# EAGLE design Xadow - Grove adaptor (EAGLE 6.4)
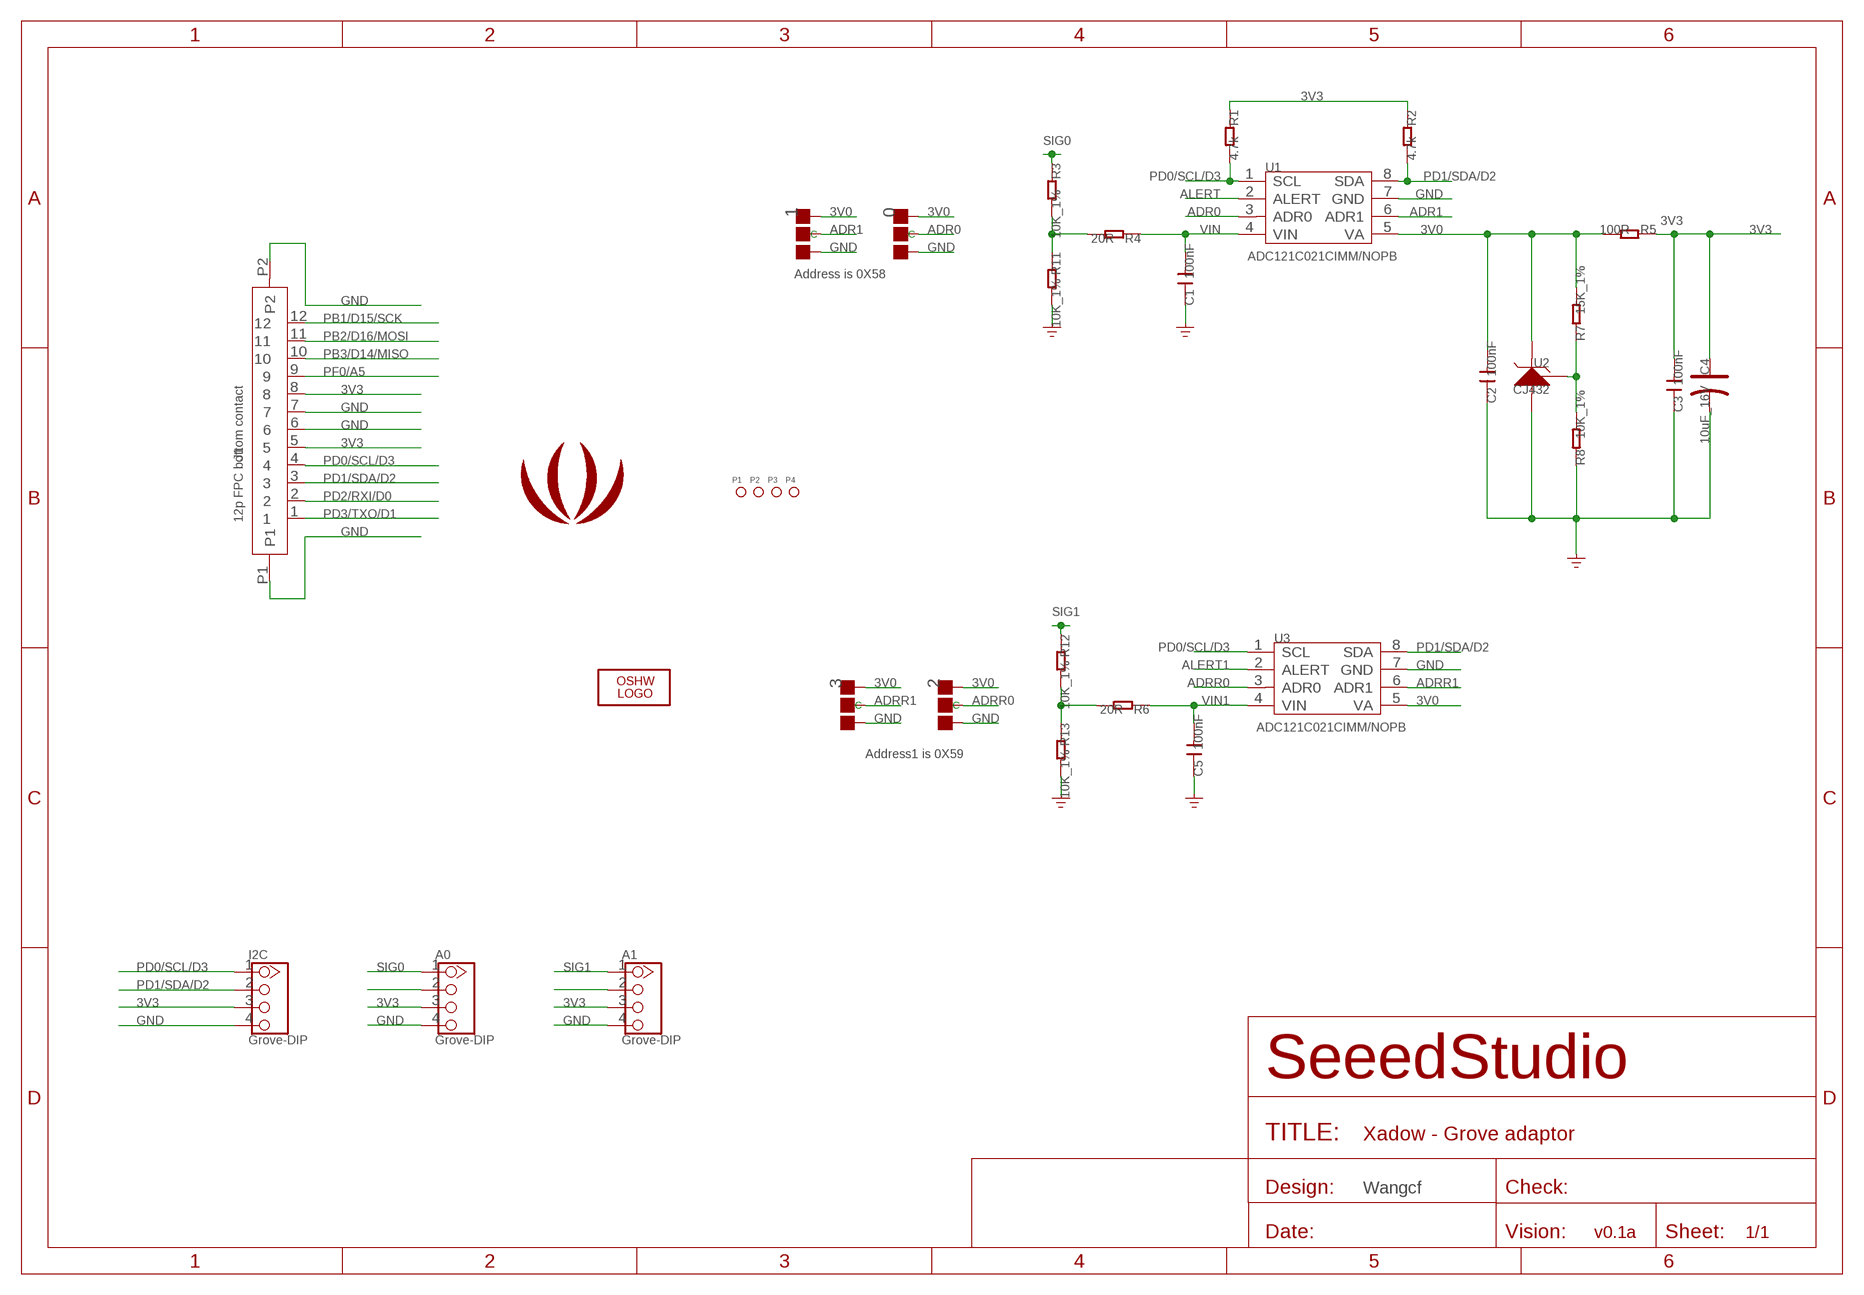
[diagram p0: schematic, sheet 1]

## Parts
0  DNP  PAD-JUMPER-3P-40*40  [3P-SMD-4.1X1.5]
1  DNP  PAD-JUMPER-3P-40*40  [3P-SMD-4.1X1.5]
2  DNP  PAD-JUMPER-3P-40*40  [3P-SMD-4.1X1.5]
3  DNP  PAD-JUMPER-3P-40*40  [3P-SMD-4.1X1.5]
A0  Grove-DIP  TWIG-2.0-LEADED  [4P-LEADED-2.0]
A1  Grove-DIP  TWIG-2.0-LEADED  [4P-LEADED-2.0]
C1  100nF  C-0603  [C0603]
C2  100nF  C-0603  [C0603]
C3  100nF  C-0603  [C0603]
C4  10uF_16V  CAP-AVX-A  [AVX-A]
C5  100nF  C-0603  [C0603]
I2C  Grove-DIP  TWIG-2.0-LEADED  [4P-LEADED-2.0]
J1  12p FPC bottom contact  FPC052002-12LT  [12P-0.5]
LOGO2  LOGO-OSHW-FILLX0100-NT  [OSHW_FILLX100_NOTEXT]
P1  PAD-MARK  [ROUND-MARK-1.0]
P2  PAD-MARK  [ROUND-MARK-1.0]
P3  PAD-MARK  [ROUND-MARK-1.0]
P4  PAD-MARK  [ROUND-MARK-1.0]
R1  4.7k  R-0603  [R0603]
R2  4.7k  R-0603  [R0603]
R3  10K_1%  R-0603  [R0603]
R4  20R  R-0603  [R0603]
R5  100R  R-0603  [R0603]
R6  20R  R-0603  [R0603]
R7  15K_1%  R-0603  [R0603]
R8  10K_1%  R-0603  [R0603]
R11  10K_1%  R-0603  [R0603]
R12  10K_1%  R-0603  [R0603]
R13  10K_1%  R-0603  [R0603]
U1  ADC121C021CIMM/NOPB  ADC121C021'CIMM/NP8'  [MSOP8]
U2  CJ432  REFERENCE-SOURCE  [SOT23]
U3  ADC121C021CIMM/NOPB  ADC121C021'CIMM/NP8'  [MSOP8]
U$7  LOGO-SEEEDSTUDIO-SMALL-SILK  [SMALL_SEEED_LOGO]

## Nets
3V0: 0.11(R) 1.11(R) 2.11(R) 3.11(R) C2.2 R5.2 R7.2 U1.5(VA) U2.2(K) U3.5(VA)
3V3: A0.3 A1.3 C3.2 C4.+ I2C.3 J1.5 J1.8 R1.1 R2.1 R5.1
ADR0: 0.MM(C) U1.3(ADR0)
ADR1: 1.MM(C) U1.6(ADR1)
ADRR0: 2.MM(C) U3.3(ADR0)
ADRR1: 3.MM(C) U3.6(ADR1)
ALERT: U1.2(ALERT)
ALERT1: U3.2(ALERT)
GND: 0.00(L) 1.00(L) 2.00(L) 3.00(L) A0.4 A1.4 C1.1 C2.1 C3.1 C4.- C5.1 I2C.4 J1.6 J1.7 J1.P1 J1.P2 R8.1 R11.2 R13.2 U1.7(GND) U2.3(A) U3.7(GND)
N$1: R7.1 R8.2 U2.1(R)
N$2: R3.2 R4.2 R11.1
N$3: R6.2 R12.2 R13.1
N$4: A0.2
N$5: A1.2
PB1/D15/SCK: J1.12
PB2/D16/MOSI: J1.11
PB3/D14/MISO: J1.10
PD0/SCL/D3: I2C.1 J1.4 R1.2 U1.1(SCL) U3.1(SCL)
PD1/SDA/D2: I2C.2 J1.3 R2.2 U1.8(SDA) U3.8(SDA)
PD2/RXI/D0: J1.2
PD3/TXO/D1: J1.1
PF0/A5: J1.9
SIG0: A0.1 R3.1
SIG1: A1.1 R12.1
VIN: C1.2 R4.1 U1.4(VIN)
VIN1: C5.2 R6.1 U3.4(VIN)

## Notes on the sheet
- 3V3
- Address is 0X58
- Address1 is 0X59
- Wangcf
- v0.1a

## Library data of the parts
0 1-3 = Discrete:PAD-JUMPER-3P; PARTNO: DNP
A0 A1 I2C = Connector:TWIG-2.0-LEADED
C1-C3 C5 = Discrete:C*: Ceramic Capacitors
C4 = Discrete1:CAP*: Electrolytic Capacitors,Tantalum Capacitors and Super Capacitors
J1 = template:FPC052002-12LT
LOGO2 = Logo:LOGO-OSHW-FILL; PARTNO: DNP
P1-P4 = Discrete:PAD-MARK; PARTNO: DNP
R1-R8 R11-R13 = Discrete:R*
U1 U3 = IC:ADC121C021: ADC121C021/ADC121C021Q/ADC121C027 I2C-Compatible, 12-Bit Analog-to-Digital Converter with Alert Function
U2 = For_Test_Albert_v6:REFERENCE-SOURCE: CJ432,AZ432 or other Adjustable Reference Source
U$7 = Logo:LOGO-SEEEDSTUDIO; PARTNO: DNP

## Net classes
0 default: width 0.152 mm, drill 0.305 mm, clearance 0.152 mm
1 GND: width 0.152 mm, drill 0.305 mm, clearance 0.152 mm to class 0, clearance 0.152 mm
3 usbvcc: width 0.203 mm, drill 0.305 mm, clearance 0.203 mm

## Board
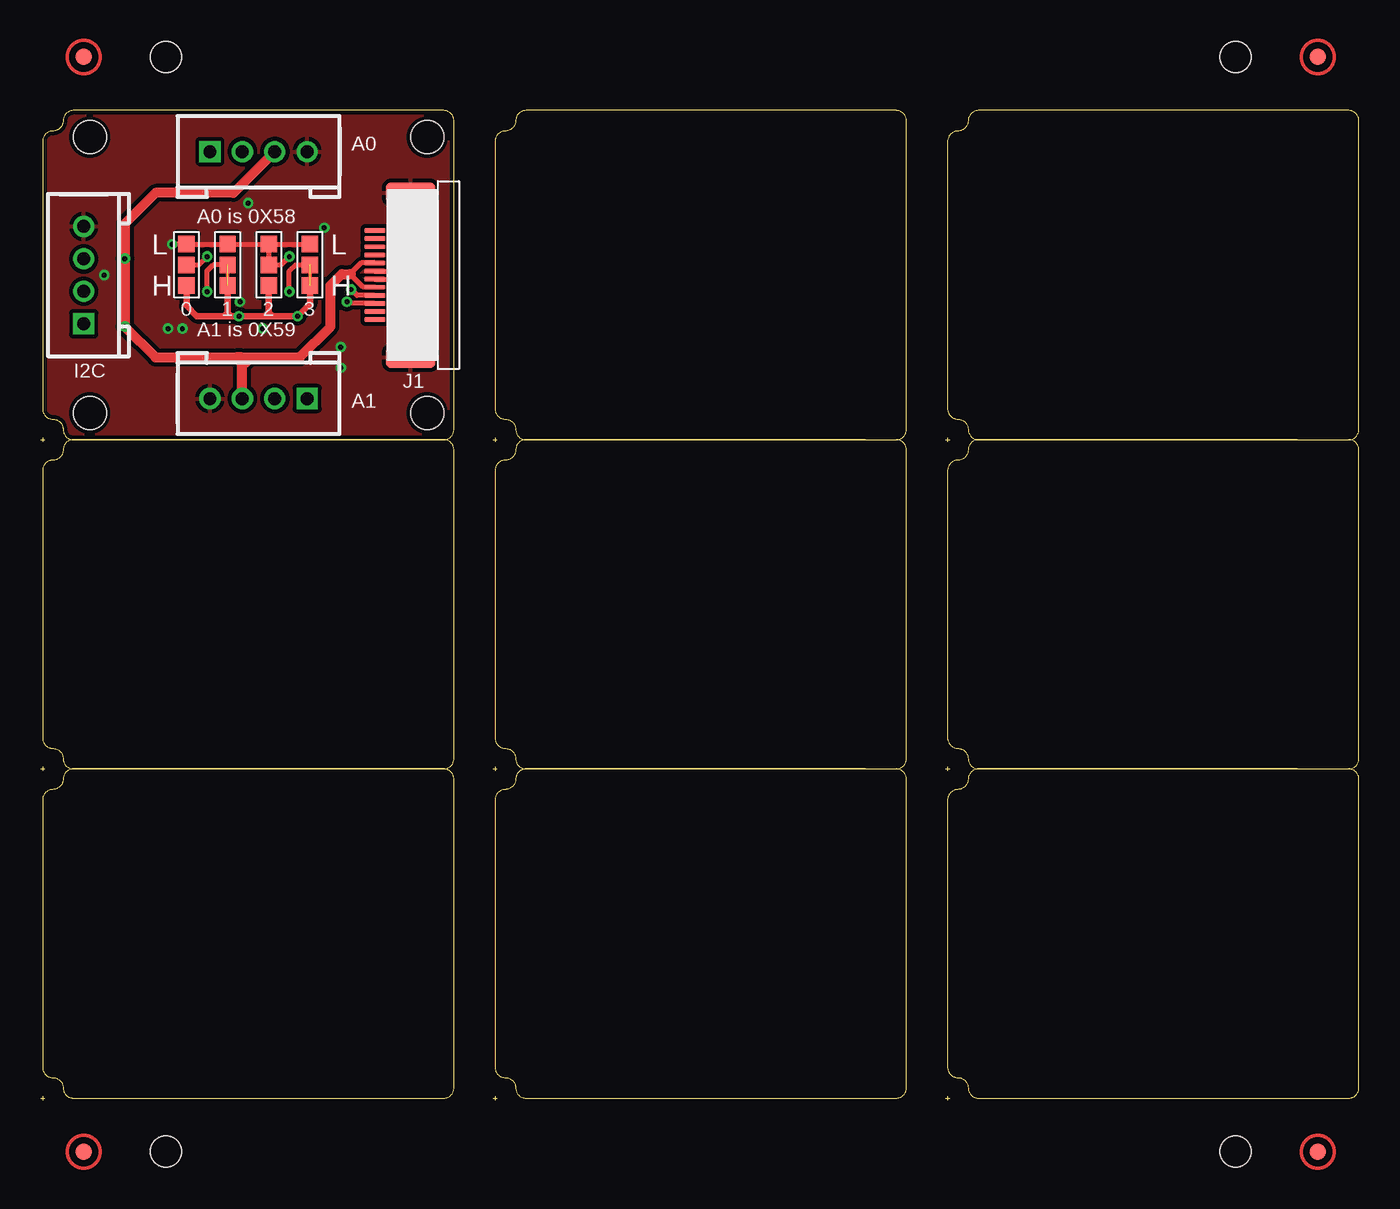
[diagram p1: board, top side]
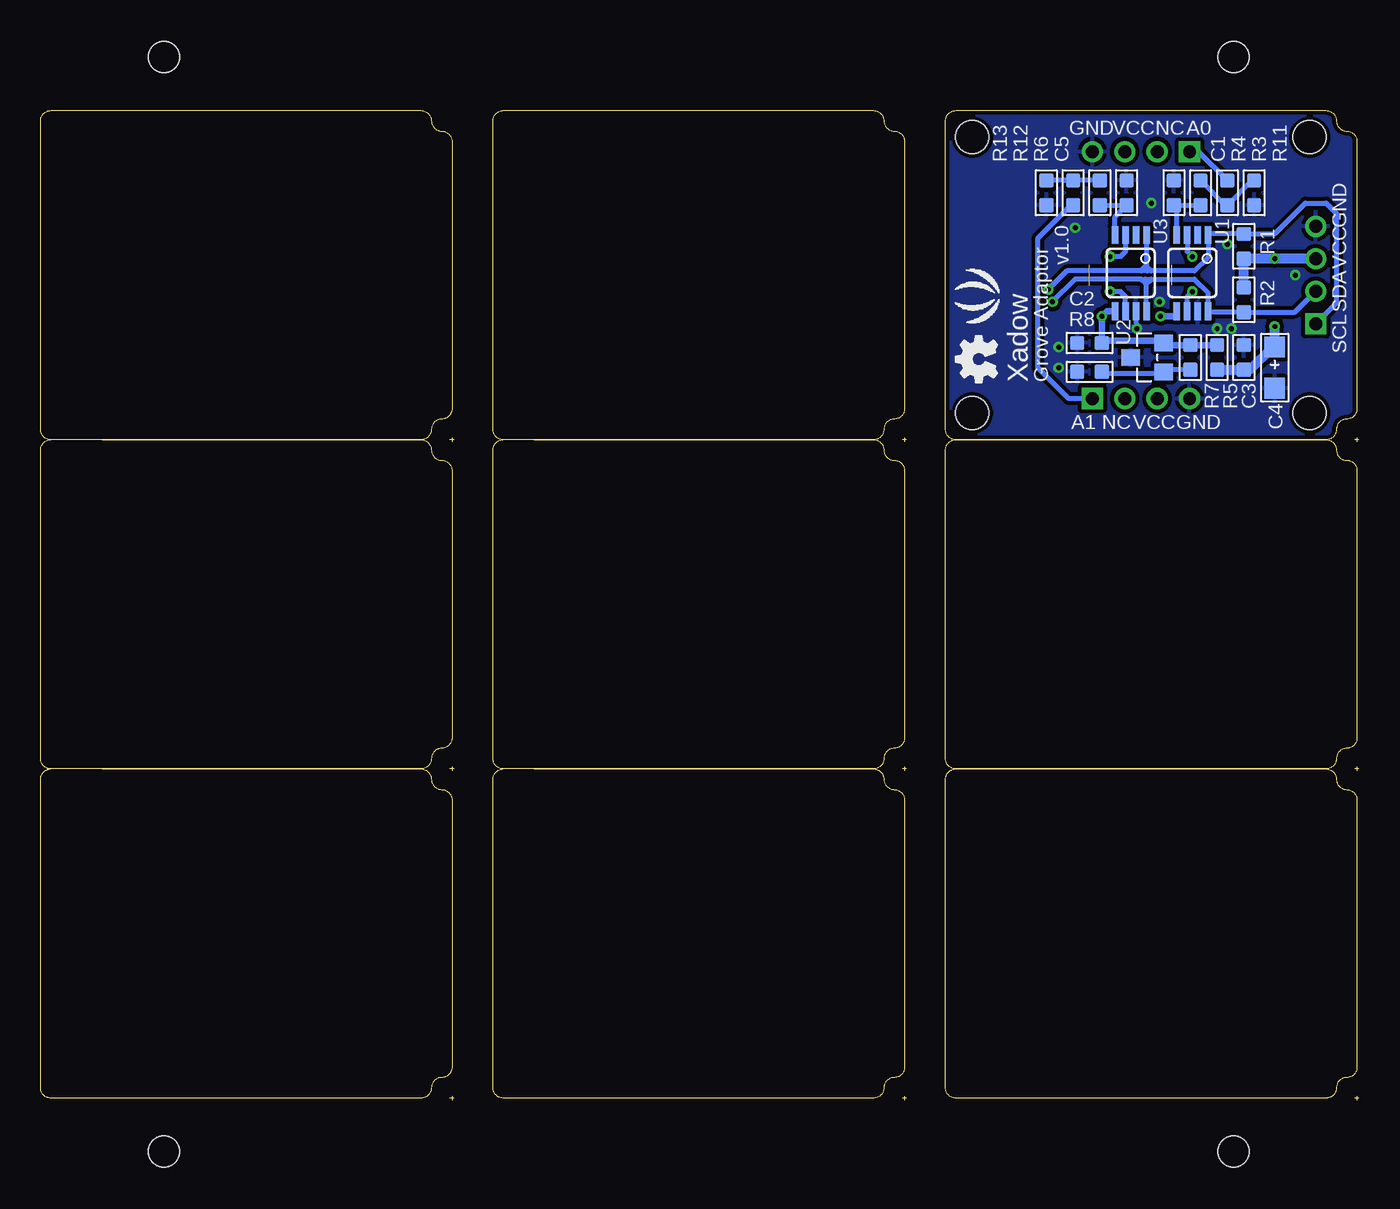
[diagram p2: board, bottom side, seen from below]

Size 81.41 x 61.09 mm. Coordinates in mm from the lower left corner, seen from the top.
Outline: 181 segments
Copper layers (1*16): Top 0.035mm / dielectric 1.5mm / Bottom 0.035mm
Design rules "SeeedStudio_rule_no_angle_090911 *": minimum track width 6mil, minimum drill 12mil, track to track 6mil, track to pad 6mil, pad to pad 6mil, via to via 6mil, smd to smd 0mil, copper to edge 10mil, drill to drill 10mil, minimum pad ring 10mil, minimum via ring 6mil, stop-mask expansion 2mil, vias tented up to drill 25mil, thermal gap 10mil
Holes 2.03 mm at 3.05,42.42 3.05,59.44 23.88,59.44 23.88,42.42
Holes 1.91 mm at 73.79,64.39 7.75,64.39 7.75,-3.17 73.79,-3.17
tRestrict: area 20.3,50.9 to 21,51

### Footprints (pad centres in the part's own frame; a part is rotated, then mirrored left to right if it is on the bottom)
3P-SMD-4.1X1.5 = smd 1.016 x 1.016: 00 -1.27,0; 11 1.27,0; MM 0,0
4P-LEADED-2.0 = drill 0.8 pad 1.27 square: 1 -3,0 | drill 0.8 pad 1.27: 2 -1,0; 3 1,0; 4 3,0
C0603 = smd 0.889 x 0.889: 1 -0.762,0; 2 0.762,0
AVX-A = smd 1.27 x 1.27: + -1.27,0; - 1.27,0
12P-0.5 = smd 0.3 x 1.3: 1 -2.75,2.35; 2 -2.25,2.35; 3 -1.75,2.35; 4 -1.25,2.35; 5 -0.75,2.35; 6 -0.25,2.35; 7 0.25,2.35; 8 0.75,2.35; 9 1.25,2.35; 10 1.75,2.35; 11 2.25,2.35; 12 2.75,2.35 | smd 1.27 x 3.048: P1 -5.08,0.127; P2 5.08,0.127
ROUND-MARK-1.0 = smd 1.016 x 1.016: P$1 0,0
R0603 = smd 0.889 x 0.889: 1 -0.762,0; 2 0.762,0
MSOP8 = smd 1.1 x 0.4: 1 -2.477,0.975; 2 -2.477,0.325; 3 -2.477,-0.325; 4 -2.477,-0.975; 5 2.223,-0.975; 6 2.223,-0.325; 7 2.223,0.325; 8 2.223,0.975
SOT23 = smd 1.016 x 1.143: 1 -0.889,-1.016; 2 0.889,-1.016; 3 0,1.016

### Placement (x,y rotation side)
0  9.02,51.56 270 top
1  11.56,51.56 270 top
2  14.1,51.56 270 top
3  16.64,51.56 270 top
A0  13.46,58.55 0 top
A1  13.46,43.31 180 top
C1  11.43,56.01 270 bottom
C2  16.64,46.74 0 bottom
C3  7.11,45.85 270 bottom
C4  5.21,45.21 270 bottom
C5  14.35,56.01 270 bottom
I2C  2.67,50.93 90 top
J1  22.99,50.93 90 top
LOGO2  22.35,44.32 90 bottom
P1  not placed on the board
P2  not placed on the board
P3  not placed on the board
P4  not placed on the board
R1  7.11,52.7 90 bottom
R2  7.11,49.4 270 bottom
R3  8.13,56.01 270 bottom
R4  9.78,56.01 90 bottom
R5  8.76,45.85 90 bottom
R6  16,56.01 90 bottom
R7  10.41,45.85 90 bottom
R8  16.64,44.96 0 bottom
R11  6.48,56.01 270 bottom
R12  17.65,56.01 90 bottom
R13  19.3,56.01 270 bottom
U1  10.29,50.93 270 bottom
U2  13.08,45.85 90 bottom
U3  14.1,50.93 270 bottom
U$7  23.75,49.66 90 bottom

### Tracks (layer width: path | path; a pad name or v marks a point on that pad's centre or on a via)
3V0  (via drill 0.3 pad 0.64)
  Top 0.305: v12.26,48.39 11.81,48.39 11.56,48.64
  Top 0.406: 3.11 16.64,49.15 v15.88,48.39 14.35,48.39 | 0.11 9.02,49.02 9.65,48.39 11.3,48.39 | 13.84,48.39 v12.26,48.39 11.56,48.39 | 14.1,48.39 14.35,48.39 | 2.11 14.1,48.64 | 14.1,48.64 14.1,48.39 | 1.11 11.56,48.64 | 11.56,48.64 11.56,48.39 | 11.56,48.64 11.3,48.39 | 11.3,48.39 11.56,48.39 | 14.1,48.64 14.35,48.39 | 14.1,48.64 13.84,48.39 | 13.84,48.39 14.1,48.39
  Bottom 0.406: R5.2 R7.2 11.94,46.61 U2.2 12.06,46.86 | U3.5 15.56,48.7 v15.88,48.39 15.88,46.86 | 15.88,46.86 C2.2 | v12.26,48.39 11.3,48.39 11.26,48.43 U1.5 | 12.06,46.99 12.06,46.86 | 12.06,46.86 15.88,46.86
3V3  (via drill 0.3 pad 0.64)
  Top 0.305: J1.5 19.93,50.18 19.3,50.8 19.3,51.18 | J1.8 19.8,51.68 19.3,51.18 | 19.3,51.18 19.11,50.99
  Top 0.61: A0.3 11.92,56.01 7.11,56.01 5.21,54.1 v5.21,51.94 v5.21,47.75 7.11,45.85 12.06,45.85 | 12.45,45.85 12.95,45.85 | A1.3 12.46,45.83 12.45,45.85 | 12.06,45.85 12.45,45.47 12.57,45.47 12.95,45.85 | 12.45,45.85 12.06,45.85 | 12.95,45.85 16,45.85 17.91,47.75 17.91,50.29 18.61,50.99 19.11,50.99
  Bottom 0.305: v5.21,51.94 R1.1
  Bottom 0.61: R5.1 C3.2 6.73,45.09 5.33,46.48 C4.+ v5.21,47.75 | R2.1 R1.1 7.1,51.93 I2C.3
ADR0  (via drill 0.3 pad 0.64)
  Top 0.305: 0.MM 9.78,51.56 v10.29,52.07
  Bottom 0.305: U1.3 10.61,52.39 v10.29,52.07
ADR1  (via drill 0.3 pad 0.64)  (1 unrouted)
  Top 0.203: 1.MM 11.56,50.29
  Top 0.305: v10.29,49.91 10.29,51.18 10.67,51.56 1.MM
  Bottom 0.305: U1.6 10.61,49.59 v10.29,49.91
ADRR0  (via drill 0.3 pad 0.64)
  Top 0.305: 2.MM 14.86,51.56 v15.37,52.07
  Bottom 0.305: U3.3 14.42,52.38 14.73,52.07 v15.37,52.07
ADRR1  (via drill 0.3 pad 0.64)  (1 unrouted)
  Top 0.203: 3.MM 16.64,50.29
  Top 0.305: v15.37,49.91 15.37,51.18 15.75,51.56 3.MM
  Bottom 0.305: U3.6 14.42,49.6 14.73,49.91 v15.37,49.91
GND  (via drill 0.3 pad 0.64)
  Top 0.305: 2.00 1.00 0.00 v8.13,52.83 | 2.00 3.00 | 2.00 14.1,51.56 | J1.7 22.35,51.18 | J1.6 22.22,50.68 22.23,50.67 22.35,50.67
  Bottom 0.305: U3.7 13.77,47.68 v13.72,47.62
  other vias: 7.87,47.62 8.76,47.62 12.83,55.37 18.54,46.48 12.32,49.28 17.53,53.85 18.54,45.21 3.94,50.93
  pour Top (isolate 0.254): 0.13,40.77 25.53,40.77 25.53,61.09 0.13,61.09
  pour Bottom (isolate 0.254): 0.13,40.77 25.53,40.77 25.53,61.09 0.13,61.09
N$1
  Bottom 0.305: R7.1 11.94,45.09 U2.1 12.06,44.83 | 12.06,44.7 12.06,44.83 | 12.06,44.83 15.75,44.83 R8.2
N$2
  Bottom 0.305: R11.1 6.73,56.77 6.73,56.64 R3.2 8.25,55.24 R4.2
N$3
  Bottom 0.305: R6.2 R12.2 | 18.29,56.77 R12.2 | R12.2 R13.1
PD0/SCL/D3  (via drill 0.3 pad 0.64)
  Top 0.305: J1.4 19.54,49.68 v19.18,50.04
  Bottom 0.305: I2C.1 1.4,49.2 1.4,54.74 2.03,55.37 3.3,55.37 5.21,53.47 R1.2 9.25,53.47 U1.1 9.31,52.03 10.16,51.18 12.83,51.18 | 13.08,51.18 13.46,51.18 | U3.1 13.12,51.52 | 13.12,51.48 13.12,51.22 13.08,51.18 | 13.12,51.52 13.46,51.18 | 13.12,51.52 13.12,51.48 | 13.12,51.48 12.83,51.18 | 12.83,51.18 13.08,51.18 | 13.46,51.18 18.03,51.18 v19.18,50.04
PD1/SDA/D2  (via drill 0.3 pad 0.64)
  Top 0.305: J1.3 19.02,49.18 v18.92,49.28
  Bottom 0.305: I2C.2 3.95,48.64 R2.2 9.25,48.64 U1.8 9.31,49.83 10.16,50.67 12.83,50.67 | 13.46,50.67 13.21,50.67 | 13.21,50.67 12.83,50.67 | U3.8 13.12,50.38 | 13.12,50.38 13.12,50.59 13.21,50.67 | 13.12,50.38 12.83,50.67 | 13.12,50.38 13.17,50.38 13.46,50.67 | 13.46,50.67 17.53,50.67 v18.92,49.28
SIG0
  Bottom 0.305: A0.1 9.91,58.55 R3.1
SIG1
  Bottom 0.305: A1.1 17.92,43.31 19.81,45.2 19.81,53.21 17.78,55.24 R12.1
VIN
  Bottom 0.305: R4.1 C1.2 11.26,55.08 U1.4
VIN1
  Bottom 0.305: U3.4 15.07,54.52 C5.2 R6.1

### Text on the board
tPlace: A0 is 0X58 | L | L | H | H | A1 is 0X59
bPlace: A0 | NC | VCC | GND | GND | v1.0 | VCC | SDA | SCL | Grove Adaptor | Xadow | GND | VCC | NC | A1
